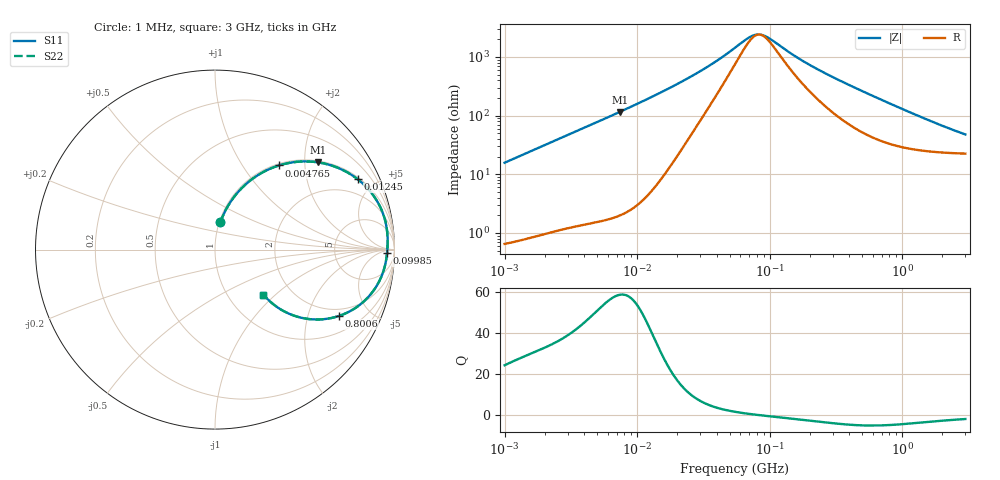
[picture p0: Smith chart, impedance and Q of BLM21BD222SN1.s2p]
! BLM21BD222SN1
# Hz S RI R 50
!Freq.(Hz) S11(Real) S11(Imag) S21(Real) S21(Imag) S12(Real) S12(Imag) S22(Real) S22(Imag)
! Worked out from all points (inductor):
!   401 points, 1 MHz to 3 GHz, reference 50 ohm
!   read as one part in series: L = 2.5 uH near 1.041 MHz
!   highest Q = 58.5 at 7.401 MHz (marker M1), where L = 2.49 uH
!   self-resonance near 84.06 MHz
!   S11 on the Smith chart (normalised r, x): 1 MHz: 1.01, +0.31; 4.765 MHz: 1.03, +1.48; 12.45 MHz: 1.10, +4.02; 99.85 MHz: 38, -19; 800.6 MHz: 1.66, -3.18; 3 GHz: 1.45, -0.84
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1000000  0.0301 0.1515  0.9699 -0.1515  0.9699 -0.1515  0.0301 0.1515
2097170  0.1039 0.2905  0.8961 -0.2905  0.8961 -0.2905  0.1039 0.2905
2831560  0.1691 0.3618  0.8309 -0.3618  0.8309 -0.3618  0.1691 0.3618
3823119  0.2654 0.4303  0.7346 -0.4303  0.7346 -0.4303  0.2654 0.4303
4764734  0.3568 0.4691  0.6432 -0.4691  0.6432 -0.4691  0.3568 0.4691
7400828  0.5719 0.4863  0.4281 -0.4863  0.4281 -0.4863  0.5719 0.4863
1.245355e7  0.7959 0.3914  0.2041 -0.3914  0.2041 -0.3914  0.7959 0.3914
1.461624e7  0.8444 0.3474  0.1556 -0.3474  0.1556 -0.3474  0.8444 0.3474
2.013356e7  0.9105 0.2573  0.0895 -0.2573  0.0895 -0.2573  0.9105 0.2573
2.944989e7  0.9478 0.1634  0.0522 -0.1634  0.0522 -0.1634  0.9478 0.1634
5.477226e7  0.9618 0.0549  0.0382 -0.0549  0.0382 -0.0549  0.9618 0.0549
6.826239e7  0.9616 0.0257  0.0384 -0.0257  0.0384 -0.0257  0.9616 0.0257
7.697298e7  0.9609 0.0107  0.0391 -0.0107  0.0391 -0.0107  0.9609 0.0107
8.679508e7  0.96 -0.00388  0.04 0.00388  0.04 0.00388  0.96 -0.00388
9.984923e7  0.9586 -0.0208  0.0414 0.0208  0.0414 0.0208  0.9586 -0.0208
1.520175e8  0.9505 -0.0742  0.0495 0.0742  0.0495 0.0742  0.9505 -0.0742
2.094008e8  0.9379 -0.1214  0.0621 0.1214  0.0621 0.1214  0.9379 -0.1214
4.304467e8  0.8603 -0.2574  0.1397 0.2574  0.1397 0.2574  0.8603 -0.2574
8.005644e8  0.6902 -0.3699  0.3098 0.3699  0.3098 0.3699  0.6902 -0.3699
1.402151e9  0.4749 -0.3783  0.5251 0.3783  0.5251 0.3783  0.4749 -0.3783
2.092429e9  0.3463 -0.3204  0.6537 0.3204  0.6537 0.3204  0.3463 -0.3204
3e9  0.2701 -0.2511  0.7299 0.2511  0.7299 0.2511  0.2701 -0.2511
